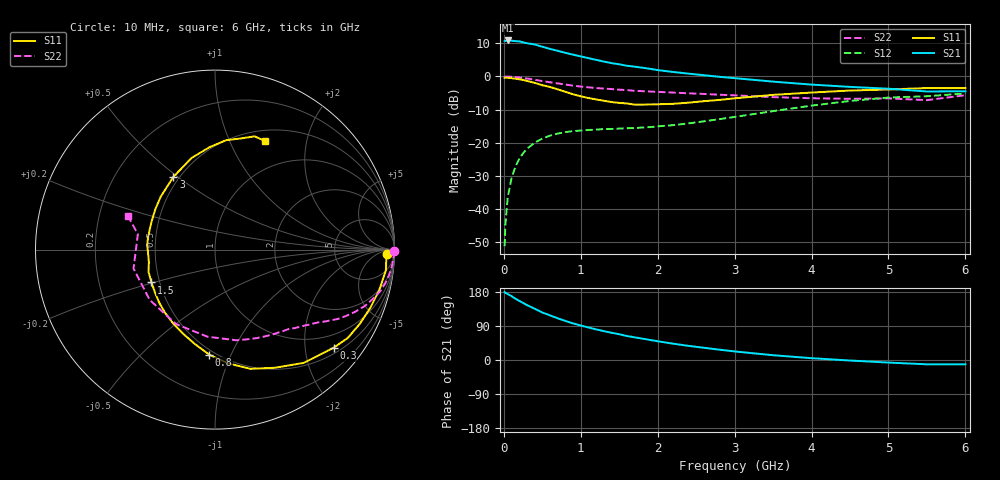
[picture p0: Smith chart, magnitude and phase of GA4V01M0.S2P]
! Infineon Technologies  Discrete & RF Semiconductors
! BF775
! Si NPN RF Bipolar Junction Transistor in SOT23
! VCE = 4 V  IC = 1 mA
! Common Emitter S-Parameters:  May  1996
# GHz  S  MA  R  50
!  f  S11  S21  S12  S22
! GHz  MAG  ANG  MAG  ANG  MAG  ANG  MAG  ANG
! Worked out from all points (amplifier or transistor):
!   36 points, 10 MHz to 6 GHz, reference 50 ohm
!   highest |S21| = 10.9 dB at 50 MHz (marker M1)
!   |S21| within 3 dB of that: start of sweep to 676.6 MHz
!   unconditionally stable (mu >= 1): 1.443 GHz to 3.971 GHz; 5.082 GHz to end of sweep
!   at 250 MHz: K = 0.20, MSG = 16.8 dB, |S12| = -23.3 dB
!   at 1.4 GHz: K = 0.98, MSG = 10.0 dB, |S12| = -15.9 dB
!   at 6 GHz: K = 1.02, MAG = -0.5 dB, |S12| = -5.1 dB
!   S11 on the Smith chart (normalised r, x): 10 MHz: 35, -20; 300 MHz: 0.64, -2.64; 800 MHz: 0.47, -0.83; 1.5 GHz: 0.45, -0.20; 3 GHz: 0.46, +0.48; 6 GHz: 0.63, +1.37
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0.01  0.958 -1.4  3.464 179.2  0.0027 89.0  0.9999 -0.5
0.02  0.9558 -2.8  3.434 177.5  0.0057 85.7  0.9954 -1.1
0.05  0.9592 -6.9  3.511 174.1  0.0146 85.8  0.9957 -2.9
0.1  0.9427 -13.7  3.484 168.5  0.029 81.8  0.9888 -5.8
0.15  0.9244 -20.5  3.427 161.7  0.0432 76.9  0.9791 -8.6
0.2  0.9068 -27.1  3.408 156.1  0.0564 73.5  0.9668 -11.3
0.3  0.8578 -39.6  3.188 145.0  0.0803 66.0  0.9334 -16.1
0.4  0.8019 -51.9  3.054 135.4  0.0995 59.2  0.8936 -20.5
0.5  0.7381 -63.1  2.823 125.4  0.1148 53.4  0.8522 -24.1
0.7  0.6394 -83.1  2.447 110.1  0.1365 44.9  0.7867 -29.4
0.8  0.5865 -93.1  2.28 103.0  0.144 41.7  0.7554 -31.5
0.9  0.5376 -102.1  2.141 96.6  0.1489 39.2  0.7273 -33.5
1.1  0.4719 -119.9  1.895 85.8  0.1549 36.0  0.6845 -37.0
1.5  0.3984 -152.7  1.529 68.0  0.1626 33.6  0.6314 -43.3
1.8  0.3738 -177.8  1.358 56.4  0.1689 35.6  0.5996 -48.0
2.2  0.3857 156.9  1.171 43.1  0.1834 39.2  0.5713 -55.9
3  0.4672 119.7  0.944 22.6  0.2442 43.9  0.5182 -77.0
3.5  0.527 104.3  0.836 12.6  0.299 42.4  0.4871 -95.0
4.5  0.6127 84.2  0.696 -1.4  0.4265 31.3  0.4592 -142.4
5  0.6353 77.0  0.653 -6.8  0.4799 23.3  0.466 -166.9
5.5  0.6687 70.7  0.593 -11.4  0.5024 14.0  0.4383 168.7
6  0.6656 65.0  0.597 -11.5  0.5541 9.2  0.5204 158.8
